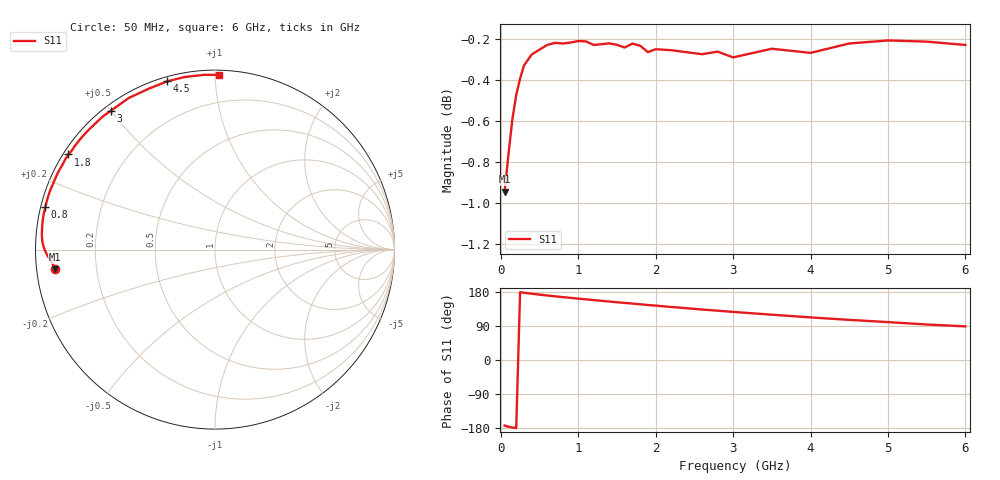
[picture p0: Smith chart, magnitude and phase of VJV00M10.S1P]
! Infineon Technologies  Discrete & RF Semiconductors
! BB 914
! Si Tuning Diode in SOT23
! VR =
! S-Parameters:  July  1999
# GHz  S  MA  R  50
!  f  S11
! GHz  MAG  ANG
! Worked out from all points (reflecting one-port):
!   34 points, 50 MHz to 6 GHz, reference 50 ohm
!   lowest |S11| = -0.9 dB at 50 MHz (marker M1), VSWR 18.42, Z = 2.73 - j3.09 ohm
!   phase of S11 starts at -173 deg and turns -98 deg over the sweep
!   S11 on the Smith chart (normalised r, x): 50 MHz: 0.05, -0.06; 800 MHz: 0.01, +0.12; 1.8 GHz: 0.01, +0.30; 3 GHz: 0.02, +0.50; 4.5 GHz: 0.02, +0.75; 6 GHz: 0.03, +1.02
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0.05  0.897 -172.9
0.1  0.916 -176.2
0.15  0.934 -177.9
0.2  0.9469 -179.6
0.3  0.9626 177.5
0.4  0.9686 174.9
0.5  0.9712 172.5
0.6  0.9738 170.3
0.8  0.9746 166.0
1  0.9759 162.0
1.1  0.9757 160.1
1.4  0.9746 154.3
1.6  0.9724 150.6
1.7  0.9745 148.9
1.8  0.9734 147.0
1.9  0.9698 145.1
2  0.9714 143.5
2.2  0.9709 139.9
2.4  0.9698 136.7
2.6  0.9688 133.2
2.8  0.9701 130.2
3  0.967 126.9
3.5  0.9717 119.6
4  0.9694 112.4
4.5  0.9746 105.9
5  0.9762 100.0
5.5  0.9756 93.7
6  0.9738 88.7
